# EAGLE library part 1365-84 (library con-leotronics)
DUAL ROW STRAIGHT HEADER 1364 SERIES. 1.27mm x 1.27mm. Without Fixing Post. SMT Source: http://www.leotronics.co.uk/Conexcon/Data%20Sheets/sec.%20A/1364ing.pdf
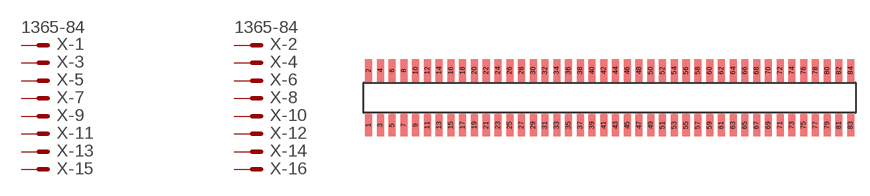
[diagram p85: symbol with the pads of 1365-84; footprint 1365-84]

Designator prefix X; gates -1=MVAL -2=MVAL -3=M -4=M -5=M -6=M -7=M -8=M -9=M -10=M -11=M -12=M -13=M -14=M -15=M -16=M -17=M -18=M -19=M -20=M -21=M -22=M -23=M -24=M -25=M -26=M -27=M -28=M -29=M -30=M -31=M -32=M -33=M -34=M -35=M -36=M -37=M -38=M -39=M -40=M -41=M -42=M -43=M -44=M -45=M -46=M -47=M -48=M -49=M -50=M -51=M -52=M -53=M -54=M -55=M -56=M -57=M -58=M -59=M -60=M -61=M -62=M -63=M -64=M -65=M -66=M -67=M -68=M -69=M -70=M -71=M -72=M -73=M -74=M -75=M -76=M -77=M -78=M -79=M -80=M -81=M -82=M -83=M -84=M

## 1365-84 (OC_FARNELL: unknown; OC_NEWARK: unknown)  [1365-84]
1  -1:S  pas
2  -2:S  pas
3  -3:S  pas
4  -4:S  pas
5  -5:S  pas
6  -6:S  pas
7  -7:S  pas
8  -8:S  pas
9  -9:S  pas
10  -10:S  pas
11  -11:S  pas
12  -12:S  pas
13  -13:S  pas
14  -14:S  pas
15  -15:S  pas
16  -16:S  pas
17  -17:S  pas
18  -18:S  pas
19  -19:S  pas
20  -20:S  pas
21  -21:S  pas
22  -22:S  pas
23  -23:S  pas
24  -24:S  pas
25  -25:S  pas
26  -26:S  pas
27  -27:S  pas
28  -28:S  pas
29  -29:S  pas
30  -30:S  pas
31  -31:S  pas
32  -32:S  pas
33  -33:S  pas
34  -34:S  pas
35  -35:S  pas
36  -36:S  pas
37  -37:S  pas
38  -38:S  pas
39  -39:S  pas
40  -40:S  pas
41  -41:S  pas
42  -42:S  pas
43  -43:S  pas
44  -44:S  pas
45  -45:S  pas
46  -46:S  pas
47  -47:S  pas
48  -48:S  pas
49  -49:S  pas
50  -50:S  pas
51  -51:S  pas
52  -52:S  pas
53  -53:S  pas
54  -54:S  pas
55  -55:S  pas
56  -56:S  pas
57  -57:S  pas
58  -58:S  pas
59  -59:S  pas
60  -60:S  pas
61  -61:S  pas
62  -62:S  pas
63  -63:S  pas
64  -64:S  pas
65  -65:S  pas
66  -66:S  pas
67  -67:S  pas
68  -68:S  pas
69  -69:S  pas
70  -70:S  pas
71  -71:S  pas
72  -72:S  pas
73  -73:S  pas
74  -74:S  pas
75  -75:S  pas
76  -76:S  pas
77  -77:S  pas
78  -78:S  pas
79  -79:S  pas
80  -80:S  pas
81  -81:S  pas
82  -82:S  pas
83  -83:S  pas
84  -84:S  pas

## Footprint 1365-84 (pad centres in mm)
DUAL ROW STRAIGHT HEADER 1364 SERIES. 1.27mm x 1.27mm. Without Fixing Post. SMT Source: http://www.leotronics.co.uk/Conexcon/Data%20Sheets/sec.%20A/1364ing.pdf
smd 0.76 x 2.4: 1 -26.035,-2.95; 2 -26.035,2.95; 3 -24.765,-2.95; 4 -24.765,2.95; 5 -23.495,-2.95; 6 -23.495,2.95; 7 -22.225,-2.95; 8 -22.225,2.95; 9 -20.955,-2.95; 10 -20.955,2.95; 11 -19.685,-2.95; 12 -19.685,2.95; 13 -18.415,-2.95; 14 -18.415,2.95; 15 -17.145,-2.95; 16 -17.145,2.95; 17 -15.875,-2.95; 18 -15.875,2.95; 19 -14.605,-2.95; 20 -14.605,2.95; 21 -13.335,-2.95; 22 -13.335,2.95; 23 -12.065,-2.95; 24 -12.065,2.95; 25 -10.795,-2.95; 26 -10.795,2.95; 27 -9.525,-2.95; 28 -9.525,2.95; 29 -8.255,-2.95; 30 -8.255,2.95; 31 -6.985,-2.95; 32 -6.985,2.95; 33 -5.715,-2.95; 34 -5.715,2.95; 35 -4.445,-2.95; 36 -4.445,2.95; 37 -3.175,-2.95; 38 -3.175,2.95; 39 -1.905,-2.95; 40 -1.905,2.95; 41 -0.635,-2.95; 42 -0.635,2.95; 43 0.635,-2.95; 44 0.635,2.95; 45 1.905,-2.95; 46 1.905,2.95; 47 3.175,-2.95; 48 3.175,2.95; 49 4.445,-2.95; 50 4.445,2.95; 51 5.715,-2.95; 52 5.715,2.95; 53 6.985,-2.95; 54 6.985,2.95; 55 8.255,-2.95; 56 8.255,2.95; 57 9.525,-2.95; 58 9.525,2.95; 59 10.795,-2.95; 60 10.795,2.95; 61 12.065,-2.95; 62 12.065,2.95; 63 13.335,-2.95; 64 13.335,2.95; 65 14.605,-2.95; 66 14.605,2.95; 67 15.875,-2.95; 68 15.875,2.95; 69 17.145,-2.95; 70 17.145,2.95; 71 18.415,-2.95; 72 18.415,2.95; 73 19.685,-2.95; 74 19.685,2.95; 75 20.955,-2.95; 76 20.955,2.95; 77 22.225,-2.95; 78 22.225,2.95; 79 23.495,-2.95; 80 23.495,2.95; 81 24.765,-2.95; 82 24.765,2.95; 83 26.035,-2.95; 84 26.035,2.95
